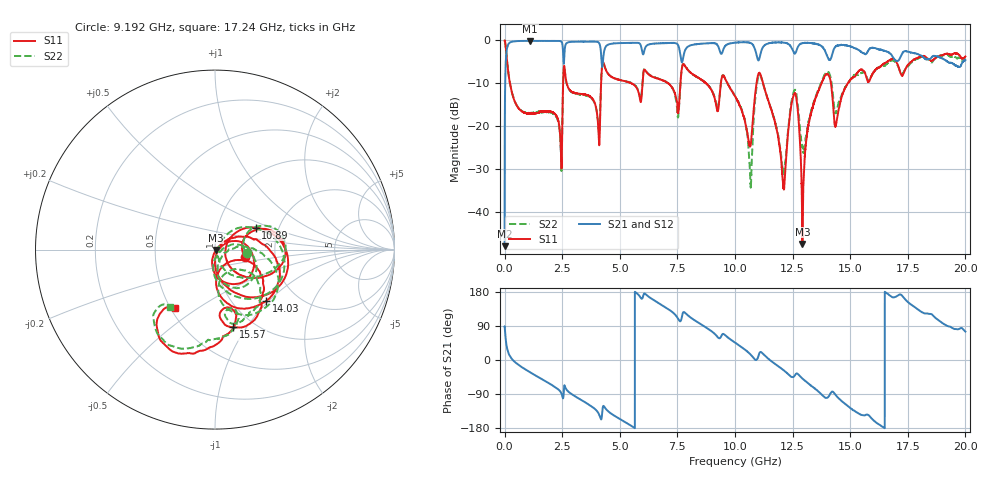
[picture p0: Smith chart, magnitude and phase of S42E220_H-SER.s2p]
!{S42E220}
!Johanson Technology Inc.
!www.johansontechnology.com
!Test Board Conditions:
!Substrate Type  RO4350B
!Substrate Thickness  50 mil
!Substrate Dk  3.66
!TL Type: GCPW
!TL Trace Width  60 mil
!TL Gap  10 mil
!Electrode orientation  Horizontal
!DUT TOPOLOGY	SERIES
!Mounting Pad LxW  14x55 mil
! Created Wed Nov 25 22:06:29 2020
# khz S ma R 50
! 2 Port Network Data from SP1.SP block
! freq  magS11  angS11  magS21  angS21  magS12  angS12  magS22  angS22
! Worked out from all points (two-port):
!   20001 points, 300 kHz to 20 GHz, reference 50 ohm
!   highest |S21| = -0.10 dB at 1.105 GHz (marker M1); lowest = -47.9 dB at 300 kHz (marker M2)
!   |S21| within 3 dB of the highest: 73.08 MHz to 2.541 GHz (2.468 GHz wide, 189 % of centre); 11.11 GHz to 13.96 GHz (2.85 GHz wide, 22.7 % of centre)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
!   lowest |S11| = -47.4 dB at 12.92 GHz (marker M3), VSWR 1.01, Z = 50.3 - j0.275 ohm
!   |S11| at or under -10 dB: 232 MHz to 2.539 GHz (2.307 GHz wide, 167 % of centre); 2.694 GHz to 4.188 GHz (1.494 GHz wide, 43.4 % of centre); 11.22 GHz to 13.76 GHz (2.537 GHz wide, 20.3 % of centre)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
!   |S22| runs from -34.3 to 0.0 dB; largest |S21 - S12| = 0.019
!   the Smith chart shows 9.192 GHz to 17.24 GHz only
!   S11 on the Smith chart (normalised r, x): 9.192 GHz: 1.39, -0.11; 10.89 GHz: 1.52, +0.40; 14.03 GHz: 1.41, -0.96; 15.57 GHz: 0.81, -0.87; 17.24 GHz: 0.53, -0.41
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300  0.9941 -0.4  0.004018 88.7  0.004025 90.2  0.9957 -0.5
147300  0.4536 -68.2  0.8876 21.7  0.8889 21.6  0.4567 -68.1
1105300  0.1406 -123.0  0.9885 -32.4  0.9867 -32.4  0.1433 -123.2
2406300  0.08346 -165.3  0.9851 -82.2  0.9845 -82.2  0.07954 -165.1
2626300  0.4102 -153.2  0.8489 -70.8  0.8499 -70.8  0.4071 -150.8
3334300  0.2377 160.3  0.9684 -105.8  0.9676 -105.8  0.2339 167.8
6667300  0.3578 64.2  0.9244 150.8  0.9222 150.7  0.3603 59.7
9192300  0.1703 -13.1  0.9122 64.4  0.9131 64.4  0.1781 -6.1
1.00003e7  0.2247 -42.2  0.9415 45.9  0.941 46.1  0.2258 -44.3
1.06623e7  0.05941 -0.8  0.9367 15.3  0.9364 15.3  0.02501 -44.7
1.08893e7  0.2578 28.4  0.7576 0.4  0.7576 0.6  0.2233 34.2
1.11413e7  0.3759 -42.8  0.7534 20.6  0.7554 20.8  0.3666 -45.7
1.21113e7  0.01931 -41.0  0.9444 -27.0  0.9454 -27.1  0.02821 -45.8
1.26083e7  0.2436 -42.5  0.7053 -39.7  0.7111 -39.9  0.2653 -44.0
1.29243e7  0.004247 -40.1  0.9308 -48.9  0.9299 -49.2  0.05812 -53.7
1.33343e7  0.153 28.4  0.9266 -69.3  0.9257 -69.1  0.161 5.8
1.40273e7  0.4039 -45.0  0.6359 -98.8  0.6372 -98.7  0.4286 -48.5
1.43813e7  0.1045 -42.3  0.8571 -93.2  0.8569 -93.1  0.1455 -52.8
1.55703e7  0.4447 -76.8  0.7109 -145.7  0.718 -146.1  0.4272 -70.5
1.66673e7  0.5759 -99.5  0.7268 172.9  0.7112 172.7  0.5582 -102.7
1.72363e7  0.3917 -124.0  0.6906 170.9  0.6832 170.8  0.4051 -127.5
2e7  0.6522 162.1  0.5883 75.0  0.5859 76.0  0.6346 162.5
